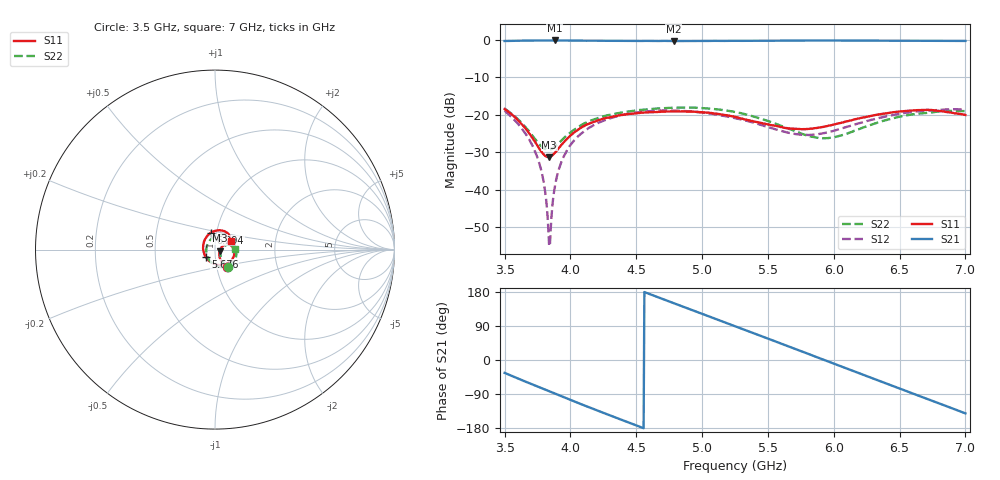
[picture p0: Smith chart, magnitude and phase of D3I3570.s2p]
! 11/4/2020 1:07:21 PM
! C:\USERS\DITOM\DESKTOP\SINGLE JUNCTION ISOLATOR DATA\3.5-7.0 GHZ (D3I3570).S2P
! CHANNEL.1
! TR.MEASUREMENT
! CORRECTED.DATA
# GHZ S RI R 50.0
! FREQ.GHZ  S11RE  S11IM  S21RE  S21IM  S12RE  S12IM  S22RE  S22IM
!; PortSelection: Port_12
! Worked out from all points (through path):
!   601 points, 3.5 GHz to 7 GHz, reference 50 ohm
!   highest |S21| = -0.16 dB at 3.879 GHz (marker M1); lowest = -0.3 dB at 4.783 GHz (marker M2)
!   lowest |S11| = -31.3 dB at 3.838 GHz (marker M3), VSWR 1.06, Z = 52.7 - j0.62 ohm
!   |S11| at or under -10 dB: start of sweep to end of sweep
!   |S22| runs from -29.4 to -18.1 dB; largest |S21 - S12| = 1.1
!   S11 on the Smith chart (normalised r, x): 3.5 GHz: 1.12, -0.22; 5.676 GHz: 0.90, -0.07; 6.294 GHz: 0.94, +0.18; 7 GHz: 1.19, +0.11
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3.5  0.0675 -0.098  0.8003 -0.5401  -0.1114 -0.0191  0.0736 -0.0958
3.634167  0.0349 -0.0648  0.5795 -0.7842  -0.0617 0.0179  0.0412 -0.0641
3.739167  0.0244 -0.0331  0.3561 -0.9127  -0.0244 0.0171  0.0308 -0.0331
3.791667  0.0242 -0.0181  0.2349 -0.9512  -0.0105 0.00934  0.0309 -0.0188
3.838333  0.0266 -0.00587  0.1243 -0.9735  -0.00174 -0.000223  0.0334 -0.00661
3.855833  0.028 -0.00155  0.0823 -0.9774  0.000574 -0.00426  0.0346 -0.00283
3.879167  0.0304 0.00367  0.0256 -0.9815  0.00287 -0.00993  0.037 0.00213
3.949167  0.0395 0.0165  -0.1414 -0.9697  0.00417 -0.0273  0.0464 0.0147
4.089167  0.0622 0.0291  -0.4535 -0.8661  -0.0148 -0.0555  0.0688 0.0269
4.375  0.097 0.0167  -0.8867 -0.3936  -0.0881 -0.0416  0.1051 0.0144
4.666667  0.1076 -0.0177  -0.9348 0.2407  -0.1038 0.0458  0.1194 -0.0213
4.783333  0.1052 -0.0339  -0.8366 0.4796  -0.0832 0.0772  0.1176 -0.0396
5.010833  0.0831 -0.0683  -0.4889 0.8345  -0.0208 0.1042  0.0961 -0.0756
5.25  0.0343 -0.0871  0.0167 0.9708  0.0348 0.0829  0.0489 -0.0974
5.454167  -0.0114 -0.0762  0.4498 0.8652  0.0532 0.0492  0.00149 -0.0876
5.675833  -0.0525 -0.0389  0.8167 0.5393  0.0499 0.0265  -0.0368 -0.0514
5.839167  -0.0653 -6.82e-05  0.9595 0.2002  0.0492 0.0219  -0.0486 -0.0141
6.060833  -0.0575 0.0533  0.9358 -0.2922  0.0639 0.0156  -0.038 0.0371
6.294167  -0.0211 0.095  0.6506 -0.7278  0.0845 -0.0161  0.00286 0.0745
6.416667  0.00539 0.1054  0.4227 -0.878  0.0858 -0.0445  0.0308 0.0808
6.696667  0.0655 0.0957  -0.1854 -0.9488  0.0374 -0.1067  0.0872 0.0589
7  0.0884 0.0452  -0.7501 -0.6108  -0.0605 -0.1013  0.1116 0.00524
